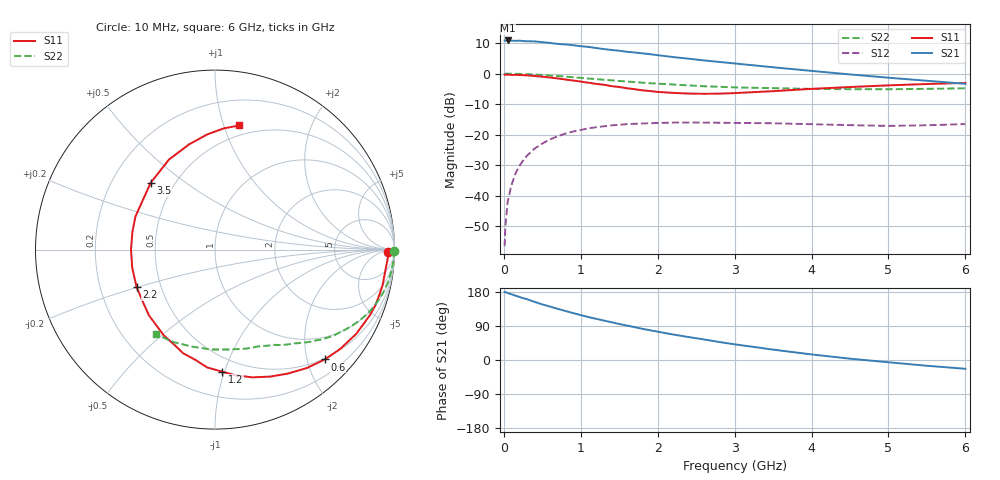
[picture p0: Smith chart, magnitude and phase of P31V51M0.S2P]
! SIEMENS Small Signal Semiconductors
! BFP181
! Si NPN RF Bipolar Junction Transistor in SOT143
! VCE = 1.5 V  IC = 1 mA
! Common Emitter S-Parameters:  March  1996
# GHz  S  MA  R  50
!  f  S11  S21  S12  S22
! GHz  MAG  ANG  MAG  ANG  MAG  ANG  MAG  ANG
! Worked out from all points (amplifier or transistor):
!   36 points, 10 MHz to 6 GHz, reference 50 ohm
!   highest |S21| = 10.9 dB at 50 MHz (marker M1)
!   |S21| within 3 dB of that: start of sweep to 1.36 GHz
!   unconditionally stable (mu >= 1): 2.98 GHz to end of sweep
!   at 250 MHz: K = 0.09, MSG = 19.6 dB, |S12| = -28.5 dB
!   at 1.4 GHz: K = 0.51, MSG = 12.3 dB, |S12| = -16.9 dB
!   at 6 GHz: K = 1.32, MAG = 3.2 dB, |S12| = -16.5 dB
!   S11 on the Smith chart (normalised r, x): 10 MHz: 44, -18; 600 MHz: 0.48, -2.33; 1.2 GHz: 0.39, -0.98; 2.2 GHz: 0.36, -0.20; 3.5 GHz: 0.37, +0.38; 6 GHz: 0.41, +1.13
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0.01  0.9618 -0.9  3.472 179.7  0.0015 89.7  0.9978 -0.3
0.02  0.9665 -1.7  3.454 179.3  0.0032 90.5  0.9965 -0.7
0.05  0.962 -3.6  3.493 176.7  0.0081 89.8  0.9969 -1.8
0.1  0.9554 -7.9  3.461 173.4  0.0151 84.8  0.9958 -3.7
0.2  0.9496 -15.5  3.466 166.6  0.0305 80.0  0.99 -7.3
0.4  0.9166 -30.7  3.37 153.3  0.0594 70.0  0.9677 -14.3
0.5  0.8911 -38.3  3.278 146.7  0.0717 64.8  0.9515 -17.6
0.6  0.8654 -45.0  3.185 141.0  0.0838 60.2  0.9342 -20.8
0.8  0.802 -59.4  3.004 129.4  0.1043 52.1  0.8951 -26.4
0.9  0.7717 -66.5  2.921 123.8  0.113 48.0  0.8731 -29.1
1.1  0.7098 -80.7  2.74 113.2  0.1271 40.8  0.8316 -33.9
1.2  0.681 -86.7  2.626 108.7  0.1328 37.2  0.8139 -36.3
1.5  0.6041 -107.1  2.374 95.1  0.1455 29.0  0.7581 -41.8
1.7  0.5567 -120.8  2.22 86.6  0.1509 24.2  0.7263 -45.3
1.9  0.5198 -134.9  2.081 78.5  0.1544 19.9  0.6973 -48.4
2.2  0.4843 -154.4  1.868 67.3  0.1581 14.5  0.6642 -52.8
2.8  0.4705 168.0  1.555 47.5  0.1573 6.2  0.6098 -61.5
3.5  0.5167 133.9  1.272 27.4  0.1541 -0.1  0.5787 -72.3
4  0.5634 117.1  1.109 14.7  0.1487 -2.7  0.5625 -81.7
4.5  0.6036 103.9  0.971 3.5  0.1435 -4.2  0.557 -92.1
5.5  0.6766 86.0  0.764 -15.2  0.1429 -1.6  0.5642 -113.8
6  0.7051 78.9  0.682 -23.2  0.1495 -0.5  0.5755 -124.9
